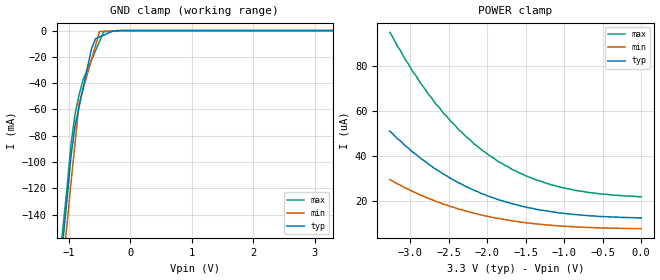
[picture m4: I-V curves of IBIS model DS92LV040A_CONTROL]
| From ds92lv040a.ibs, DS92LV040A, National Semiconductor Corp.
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[Model]   DS92LV040A_CONTROL
Model_type Input
Vinh=2.0
Vinl=0.8
C_comp   3.834p   NA   NA
[Temperature Range] 25   85   -40
[Voltage Range]   3.3   3.00   3.60
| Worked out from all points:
|   GND clamp passes 1 mA (typ) near -0.31 V on its own axis
[GND Clamp]
-3.3V     -1.36A     -1.35A     -1.39A
-1.1V     -162mA     -179mA     -152mA
-1.03V    -129mA     -148mA     -120mA
-967mV    -96.5mA    -117mA     -87.8mA
-900mV    -72.8mA    -86.2mA    -63.9mA
-833mV    -58.1mA    -55.4mA    -48.9mA
-633mV    -14.3mA    -22.6mA    -22.7mA
-567mV    -6.25mA    -11.6mA    -15.4mA
-500mV    -4.86mA    -677uA     -8.17mA
-433mV    -3.47mA    -541uA     -919uA
-100mV    -2.96uA    -229nA     -6.79nA
3.3V      910pA      1.9nA      287pA
[POWER Clamp]
-3.27V    51.2uA     29.6uA     95.1uA
-3.17V    47.8uA     27.7uA     88.9uA
-2.97V    41.8uA     24.3uA     77.6uA
-2.77V    36.6uA     21.3uA     67.7uA
-2.57V    32uA       18.6uA     59.1uA
-2.37V    28.1uA     16.5uA     51.7uA
-2.17V    24.8uA     14.6uA     45.4uA
-1.87V    20.8uA     12.4uA     37.9uA
-1.5V     17.4uA     10.4uA     31.3uA
-1.07V    14.8uA     9.01uA     26.4uA
-666mV    13.5uA     8.3uA      23.8uA
0V        12.6uA     7.79uA     22uA
